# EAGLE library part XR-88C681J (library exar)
DUAL UART full duplex
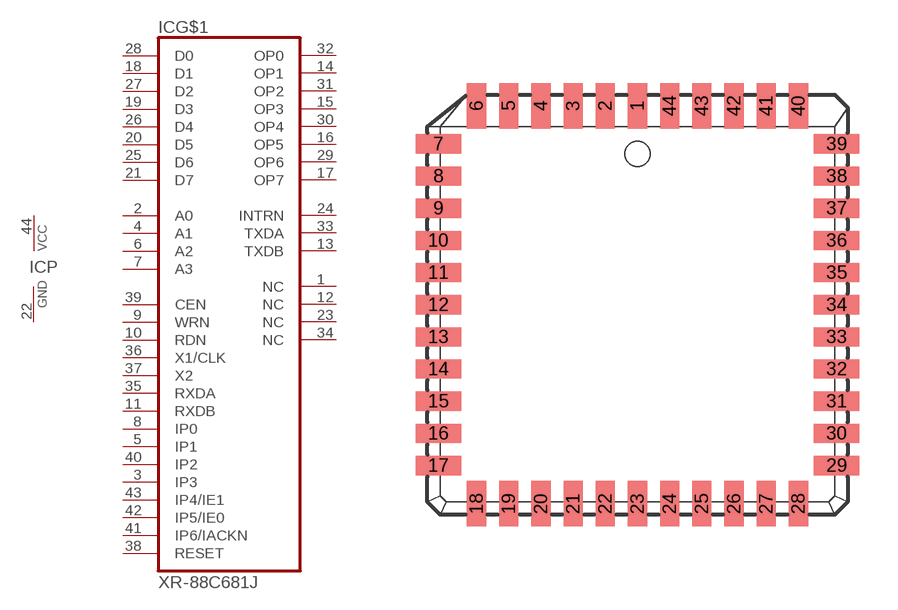
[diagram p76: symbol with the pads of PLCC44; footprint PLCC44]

Designator prefix IC; gates G$1=88C681J P=PWRN

## XR-88C681J (MPN: XR88C681J-F; OC_FARNELL: 1716912; OC_NEWARK: 24R2425)  [PLCC44]
1  G$1:NC  nc
2  G$1:A0  in
3  G$1:IP3  in
4  G$1:A1  in
5  G$1:IP1  in
6  G$1:A2  in
7  G$1:A3  in
8  G$1:IP0  in
9  G$1:WRN  in
10  G$1:RDN  in
11  G$1:RXDB  in
12  G$1:NC  nc
13  G$1:TXDB  out
14  G$1:OP1  out
15  G$1:OP3  out
16  G$1:OP5  out
17  G$1:OP7  out
18  G$1:D1
19  G$1:D3
20  G$1:D5
21  G$1:D7
22  P:GND  pwr
23  G$1:NC  nc
24  G$1:INTRN  out
25  G$1:D6
26  G$1:D4
27  G$1:D2
28  G$1:D0
29  G$1:OP6  out
30  G$1:OP4  out
31  G$1:OP2  out
32  G$1:OP0  out
33  G$1:TXDA  out
34  G$1:NC  nc
35  G$1:RXDA  in
36  G$1:X1/CLK  in
37  G$1:X2  in
38  G$1:RESET  in
39  G$1:CEN  in
40  G$1:IP2  in
41  G$1:IP6/IACKN  in
42  G$1:IP5/IE0
43  G$1:IP4/IE1  in
44  P:VCC  pwr

## Footprint PLCC44 (pad centres in mm)
Plastic Leaded Chip Carrier
smd 0.76 x 1.8: 1 0,7.86; 2 -1.27,7.86; 3 -2.54,7.86; 4 -3.81,7.86; 5 -5.08,7.86; 6 -6.35,7.86; 18 -6.35,-7.86; 19 -5.08,-7.86; 20 -3.81,-7.86; 21 -2.54,-7.86; 22 -1.27,-7.86; 23 0,-7.86; 24 1.27,-7.86; 25 2.54,-7.86; 26 3.81,-7.86; 27 5.08,-7.86; 28 6.35,-7.86; 40 6.35,7.86; 41 5.08,7.86; 42 3.81,7.86; 43 2.54,7.86; 44 1.27,7.86
smd 1.8 x 0.76: 7 -7.86,6.35; 8 -7.86,5.08; 9 -7.86,3.81; 10 -7.86,2.54; 11 -7.86,1.27; 12 -7.86,0; 13 -7.86,-1.27; 14 -7.86,-2.54; 15 -7.86,-3.81; 16 -7.86,-5.08; 17 -7.86,-6.35; 29 7.86,-6.35; 30 7.86,-5.08; 31 7.86,-3.81; 32 7.86,-2.54; 33 7.86,-1.27; 34 7.86,0; 35 7.86,1.27; 36 7.86,2.54; 37 7.86,3.81; 38 7.86,5.08; 39 7.86,6.35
